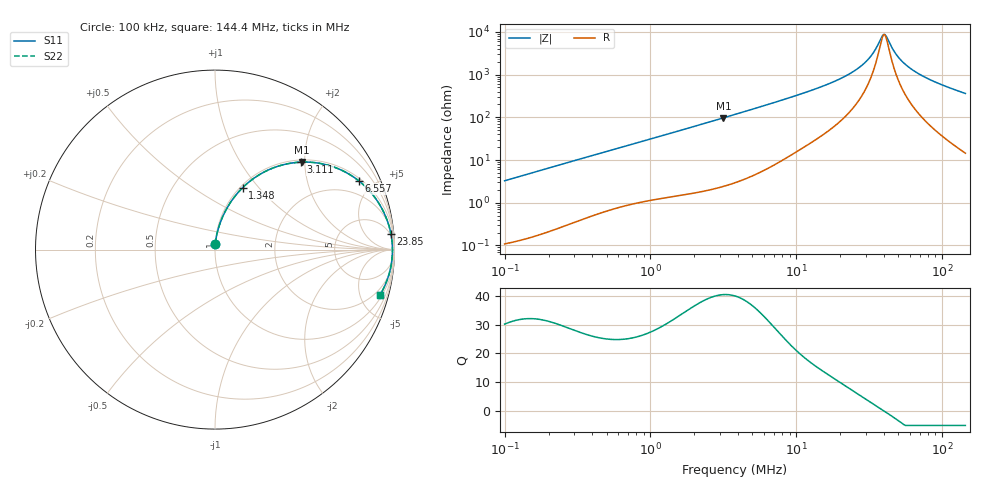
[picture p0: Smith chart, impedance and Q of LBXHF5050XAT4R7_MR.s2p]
! LBXHF5050XAT4R7_MR  S-PARAMETER MODEL  ( General Type )
! Model Generated by TAIYO YUDEN Corporation (http://www.ty-top.com)
! Version 1.0
! TAIYO YUDEN Control No. 201105NI43SB-FBB
! Copyright(c) 2020 TAIYO YUDEN CO.,LTD. All Rights Reserved.
! Product Description (link to TY-COMPAS)
! https://ds.yuden.co.jp/TYCOMPAS/or/detail?pn=LBXHF5050XAT4R7MMR&u=M
! Products Name : Inductors
! Characteristics :
!  Inductance : 4.7 uH , SRF(min) : 30 MHz , DC Resistance(max) : 0.052 Ohm
!  Rated Current : Saturation :3500 mA , Temp Rise : 1900 mA
!  Case Size : 5.0 x 5.0 / 0.197 x 0.197 [mm/inch] , Thickness : 3.1 / 0.122 [mm/inch]
!  (Conditions: Temperature = 25 degC , DC Bias Current/Voltage = 0A / 0V)
! External Node Assignments :
!  1  o---GGG---o  2
! GND o---------o GND
! Frequency Range : 0.1MHz  -  144.390904MHz  [ 402 STEP ]
# MHz S RI R 50
! Freq[MHz].  S11 Real  S11 Imag  S21 Real  S21 Imag  S12 Real  S12 Imag  S22 Real  S22 Imag
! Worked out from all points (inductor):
!   401 points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, 100 kHz to 144.4 MHz, reference 50 ohm
!   read as one part in series: L = 5.17 uH near 103.7 kHz
!   highest Q = 40.4 at 3.168 MHz (marker M1), where L = 4.88 uH
!   self-resonance near 39.69 MHz
!   S11 on the Smith chart (normalised r, x): 100 kHz: 1.00, +0.07; 1.348 MHz: 1.03, +0.83; 3.111 MHz: 1.05, +1.91; 6.557 MHz: 1.13, +4.11; 23.85 MHz: 4, +22; 144.4 MHz: 1.29, -7.24
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0.1  0.00214 0.0325  0.9979 -0.0325  0.9979 -0.0325  0.00214 0.0325
0.338238  0.0155 0.1063  0.9845 -0.1063  0.9845 -0.1063  0.0155 0.1063
1.144052  0.1194 0.3074  0.8806 -0.3074  0.8806 -0.3074  0.1194 0.3074
1.347521  0.1549 0.346  0.8451 -0.346  0.8451 -0.346  0.1549 0.346
2.010528  0.2808 0.4359  0.7192 -0.4359  0.7192 -0.4359  0.2808 0.4359
3.110875  0.4774 0.4873  0.5226 -0.4873  0.5226 -0.4873  0.4774 0.4873
3.167973  0.4863 0.4876  0.5137 -0.4876  0.5137 -0.4876  0.4863 0.4876
3.869624  0.5844 0.4804  0.4156 -0.4804  0.4156 -0.4804  0.5844 0.4804
6.557456  0.8007 0.3835  0.1993 -0.3835  0.1993 -0.3835  0.8007 0.3835
12.85266  0.938 0.2126  0.062 -0.2126  0.062 -0.2126  0.938 0.2126
18.15812  0.9676 0.1382  0.0324 -0.1382  0.0324 -0.1382  0.9676 0.1382
23.85359  0.9804 0.0868  0.0196 -0.0868  0.0196 -0.0868  0.9804 0.0868
31.33549  0.9869 0.0401  0.0131 -0.0401  0.0131 -0.0401  0.9869 0.0401
34.31869  0.988 0.0251  0.012 -0.0251  0.012 -0.0251  0.988 0.0251
38.97828  0.9887 0.00441  0.0113 -0.00441  0.0113 -0.00441  0.9887 0.00441
41.16416  0.9888 -0.00443  0.0112 0.00443  0.0112 0.00443  0.9888 -0.00443
43.47261  0.9886 -0.0133  0.0114 0.0133  0.0114 0.0133  0.9886 -0.0133
46.75318  0.9882 -0.0252  0.0118 0.0252  0.0118 0.0252  0.9882 -0.0252
51.20418  0.9873 -0.0401  0.0127 0.0401  0.0127 0.0401  0.9873 -0.0401
63.69299  0.9829 -0.0775  0.0171 0.0775  0.0171 0.0775  0.9829 -0.0775
89.98492  0.968 -0.143  0.032 0.143  0.032 0.143  0.968 -0.143
144.3909  0.9206 -0.2512  0.0794 0.2512  0.0794 0.2512  0.9206 -0.2512
